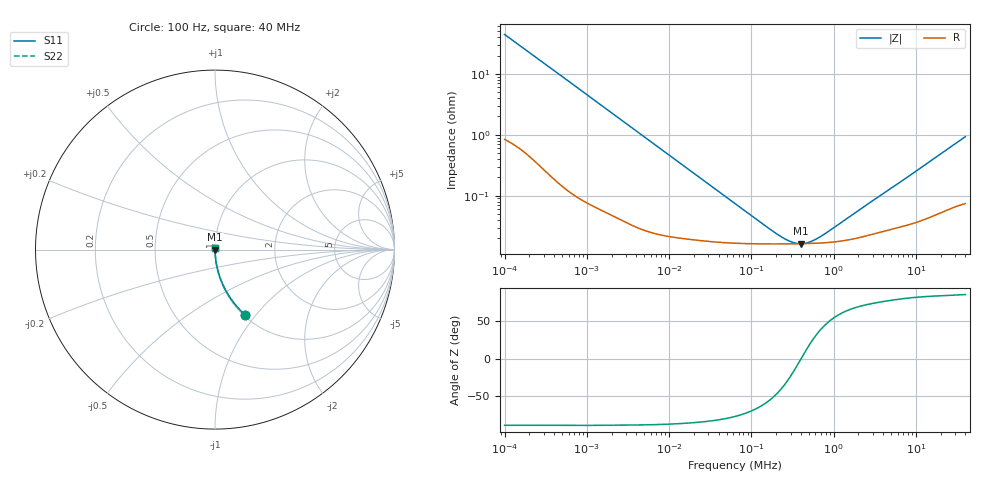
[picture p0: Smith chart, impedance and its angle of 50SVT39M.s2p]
!  *** S-Parameter ***
!  Copyright (C) Panasonic Industry
!  Conductive Polymer Aluminum Solid Capacitors (OS-CON)
!  Parts No. 50SVT39M
! Touchstone file from project
# GHZ S RI R 50.000000
! Modal data exported
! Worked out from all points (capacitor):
!   450 points, 100 Hz to 40 MHz, reference 50 ohm
!   read as one part in series: C = 35.8 uF near 105.9 Hz
!   lowest |Z| = 16.3 mohm at 398.1 kHz (marker M1)
!   series resonance near 402.5 kHz, so ESL is about 4.4 nH
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1e-07  0.1686 -0.365  0.8314 0.365  0.8314 0.365  0.1686 -0.365
1.059254e-07  0.1537 -0.3512  0.8463 0.3512  0.8463 0.3512  0.1537 -0.3512
1.496236e-07  0.0862 -0.2707  0.9138 0.2707  0.9138 0.2707  0.0862 -0.2707
2.304093e-07  0.0399 -0.1864  0.9601 0.1864  0.9601 0.1864  0.0399 -0.1864
4.216965e-07  0.013 -0.1056  0.987 0.1056  0.987 0.1056  0.013 -0.1056
8.659643e-07  0.00358 -0.0522  0.9964 0.0522  0.9964 0.0522  0.00358 -0.0522
2.113489e-06  0.000925 -0.0216  0.9991 0.0216  0.9991 0.0216  0.000925 -0.0216
7.498942e-06  0.000268 -0.00616  0.9997 0.00616  0.9997 0.00616  0.000268 -0.00616
6.493816e-05  0.000166 -0.000705  0.9998 0.000705  0.9998 0.000705  0.000166 -0.000705
0.0001584893  0.000162 -0.000251  0.9998 0.000251  0.9998 0.000251  0.000162 -0.000251
0.0002304093  0.000161 -0.000137  0.9998 0.000137  0.9998 0.000137  0.000161 -0.000137
0.0002660725  0.000162 -9.96e-05  0.9998 9.96e-05  0.9998 9.96e-05  0.000162 -9.96e-05
0.0003072557  0.000162 -6.39e-05  0.9998 6.39e-05  0.9998 6.39e-05  0.000162 -6.39e-05
0.0003548134  0.000162 -2.96e-05  0.9998 2.96e-05  0.9998 2.96e-05  0.000162 -2.96e-05
0.0003981072  0.000163 -2.57e-06  0.9998 2.57e-06  0.9998 2.57e-06  0.000163 -2.57e-06
0.000459727  0.000163 3.11e-05  0.9998 -3.11e-05  0.9998 -3.11e-05  0.000163 3.11e-05
0.0005463865  0.000164 7.24e-05  0.9998 -7.24e-05  0.9998 -7.24e-05  0.000164 7.24e-05
0.0006493816  0.000166 0.000116  0.9998 -0.000116  0.9998 -0.000116  0.000166 0.000116
0.000817523  0.000169 0.000179  0.9998 -0.000179  0.9998 -0.000179  0.000169 0.000179
0.002113489  0.000207 0.000565  0.9998 -0.000565  0.9998 -0.000565  0.000207 0.000565
0.004731513  0.000276 0.00122  0.9997 -0.00122  0.9997 -0.00122  0.000276 0.00122
0.04  0.000828 0.00927  0.9992 -0.00927  0.9992 -0.00927  0.000828 0.00927
